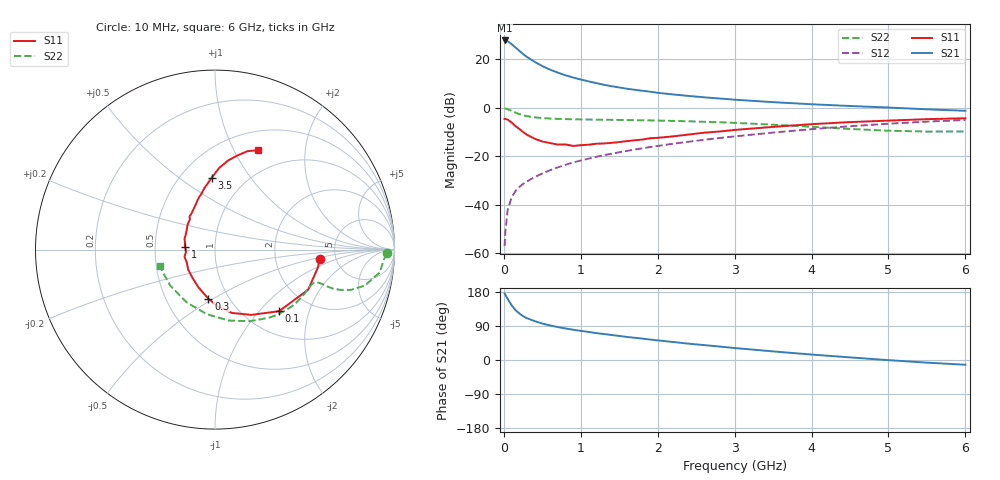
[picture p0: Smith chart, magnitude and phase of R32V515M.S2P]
! SIEMENS Small Signal Semiconductors
! BFR181
! Si NPN RF Bipolar Junction Transistor in SOT23
! VCE = 2.5 V  IC = 15 mA
! Common Emitter S-Parameters:  May  1996
# GHz  S  MA  R  50
!  f  S11  S21  S12  S22
! GHz  MAG  ANG  MAG  ANG  MAG  ANG  MAG  ANG
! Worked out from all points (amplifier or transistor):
!   36 points, 10 MHz to 6 GHz, reference 50 ohm
!   highest |S21| = 27.6 dB at 10 MHz (marker M1)
!   |S21| within 3 dB of that: start of sweep to 155.4 MHz
!   unconditionally stable (mu >= 1): 448.3 MHz to 2.747 GHz
!   at 250 MHz: K = 0.78, MSG = 26.7 dB, |S12| = -31.4 dB
!   at 1.4 GHz: K = 1.13, MAG = 11.7 dB, |S12| = -19.0 dB
!   at 6 GHz: K = 0.89, MSG = 1.9 dB, |S12| = -5.1 dB
!   S11 on the Smith chart (normalised r, x): 10 MHz: 3.72, -0.60; 100 MHz: 1.42, -1.29; 300 MHz: 0.80, -0.48; 1 GHz: 0.71, +0.02; 3.5 GHz: 0.70, +0.67; 6 GHz: 0.72, +1.25
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0.01  0.5854 -5.2  24.08 175.8  0.0014 88.6  0.9566 -1.3
0.02  0.5824 -9.7  23.8 171.8  0.0028 91.9  0.9434 -3.2
0.05  0.5651 -23.3  23.04 161.0  0.0078 78.5  0.9266 -7.9
0.1  0.495 -43.9  20.36 145.0  0.014 74.3  0.8589 -13.5
0.15  0.4167 -60.8  17.34 131.9  0.019 69.3  0.7877 -16.6
0.2  0.365 -75.1  14.81 123.1  0.0231 67.7  0.7338 -17.8
0.25  0.3145 -87.7  12.66 115.8  0.0268 67.5  0.6951 -18.3
0.3  0.2758 -97.7  11.03 110.3  0.0301 68.6  0.6644 -18.2
0.4  0.2284 -114.3  8.745 102.7  0.0372 69.2  0.6287 -17.8
0.5  0.2004 -129.1  7.14 96.2  0.0438 70.8  0.6078 -17.7
0.6  0.1862 -143.4  6.049 91.3  0.0513 71.8  0.5934 -17.8
0.7  0.1731 -155.2  5.252 87.0  0.0586 72.6  0.5843 -18.3
0.8  0.1742 -166.6  4.623 83.2  0.0662 72.5  0.5789 -18.9
1  0.1679 175.0  3.775 76.9  0.0812 73.3  0.5698 -20.5
1.1  0.1719 166.8  3.466 74.1  0.0887 72.9  0.5673 -21.6
1.3  0.1823 154.0  2.944 68.6  0.1044 72.5  0.5605 -23.7
1.6  0.2037 139.1  2.44 60.8  0.1283 71.4  0.5526 -27.6
2.2  0.2551 117.9  1.86 47.5  0.1799 68.2  0.531 -36.8
3.5  0.4001 92.7  1.292 22.7  0.3058 56.8  0.444 -64.0
4.5  0.502 81.6  1.077 6.9  0.4128 44.6  0.3624 -97.3
5.5  0.5775 71.7  0.92 -7.0  0.5129 30.2  0.3203 -140.8
6  0.6025 66.7  0.858 -12.5  0.5546 22.5  0.3224 -163.2
